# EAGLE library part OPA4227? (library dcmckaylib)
Low-noise quad op amp 8MHz bandwidth 3nv/Hz^0.5 voltage noise 0.4pA/Hz^(0.5) current noise
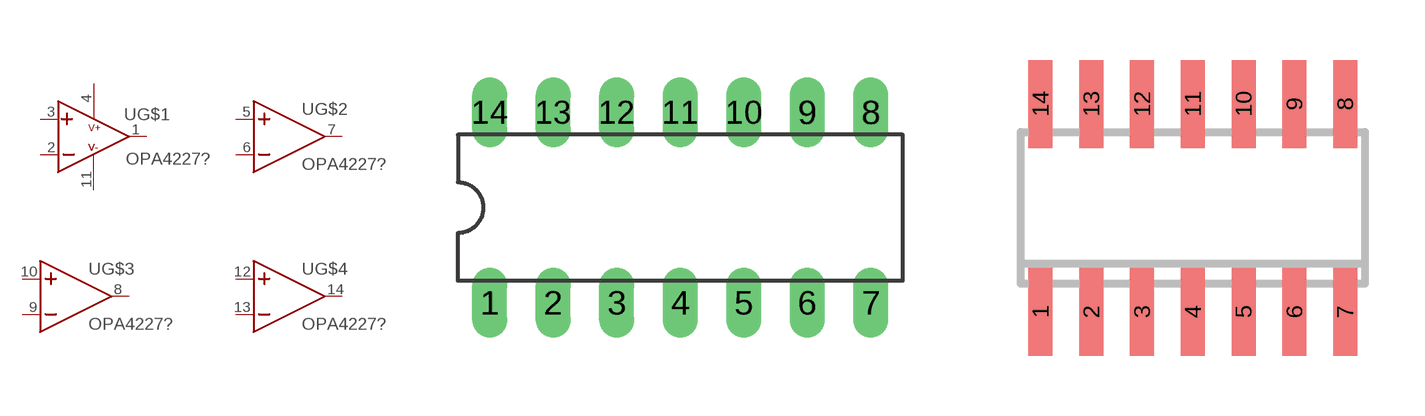
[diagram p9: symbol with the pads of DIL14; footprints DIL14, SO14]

Designator prefix U; gates G$1=OPAMP2 G$2=OPAMP G$3=OPAMP G$4=OPAMP

## OPA4227PA  [DIL14]
1  G$1:OUT  out
2  G$1:IN-  in
3  G$1:IN+  in
4  G$1:V+  pwr
5  G$2:IN+  in
6  G$2:IN-  in
7  G$2:OUT  out
8  G$3:OUT  out
9  G$3:IN-  in
10  G$3:IN+  in
11  G$1:V-  pwr
12  G$4:IN+  in
13  G$4:IN-  in
14  G$4:OUT  out

## OPA4227UA  [SO14]
Pads as for DIL14

## Footprint DIL14 (pad centres in mm)
Dual In Line Package
drill 0.889 long: 1 -7.62,-3.81; 2 -5.08,-3.81; 3 -2.54,-3.81; 4 0,-3.81; 5 2.54,-3.81; 6 5.08,-3.81; 7 7.62,-3.81; 8 7.62,3.81; 9 5.08,3.81; 10 2.54,3.81; 11 0,3.81; 12 -2.54,3.81; 13 -5.08,3.81; 14 -7.62,3.81

## Footprint SO14 (pad centres in mm)
Small Outline Package 14
smd 0.6 x 2.2: 1 -3.81,-2.6; 2 -2.54,-2.6; 3 -1.27,-2.6; 4 0,-2.6; 5 1.27,-2.6; 6 2.54,-2.6; 7 3.81,-2.6; 8 3.81,2.6; 9 2.54,2.6; 10 1.27,2.6; 11 0,2.6; 12 -1.27,2.6; 13 -2.54,2.6; 14 -3.81,2.6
